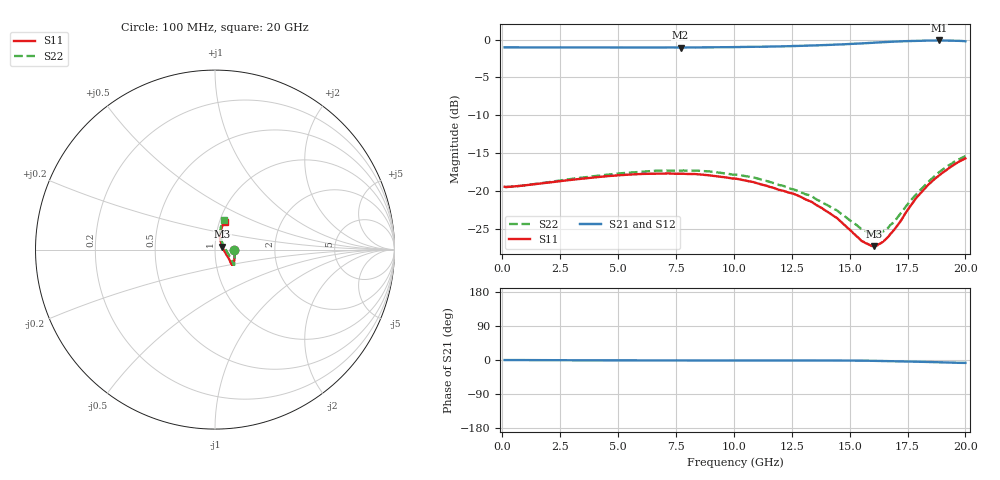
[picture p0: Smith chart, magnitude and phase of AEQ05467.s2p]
!Agilent Technologies,E8363B,MY43030965,A.07.50.67
!Agilent E8363B: A.07.50.67
!Date: Tuesday, August 27, 2013 09:58:20
!Correction: S11(Full 2 Port(1,2))
!S21(Full 2 Port(1,2))
!S12(Full 2 Port(1,2))
!S22(Full 2 Port(1,2))
!S2P File: Measurements: S11, S21, S12, S22:
# Hz S  dB  R 50
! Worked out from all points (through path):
!   3201 points, 100 MHz to 20 GHz, reference 50 ohm
!   highest |S21| = -0.11 dB at 18.86 GHz (marker M1); lowest = -1.0 dB at 7.699 GHz (marker M2)
!   lowest |S11| = -27.3 dB at 16.06 GHz (marker M3), VSWR 1.09, Z = 54.1 + j1.8 ohm
!   |S11| at or under -10 dB: start of sweep to end of sweep
!   |S22| runs from -25.7 to -15.4 dB; largest |S21 - S12| = 0.0079
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1e8  -19.44 -1.0  -1.02 -0.1  -1.02 -0.0  -19.48 -0.9
3.420812e9  -18.37 -26.0  -1.03 -0.7  -1.04 -0.8  -18.23 -26.0
5.162062e9  -17.89 -34.6  -1.04 -1.0  -1.04 -1.0  -17.64 -33.8
6.735406e9  -17.70 -39.2  -1.04 -1.2  -1.04 -1.3  -17.32 -37.7
7.699312e9  -17.71 -40.5  -1.05 -1.3  -1.06 -1.1  -17.30 -38.4
8.90575e9  -17.90 -41.5  -1.01 -1.3  -1.03 -1.2  -17.40 -38.7
1.005e10  -18.37 -40.7  -0.98 -1.3  -1.02 -1.0  -17.83 -37.5
1.098281e10  -18.95 -39.5  -0.94 -1.3  -0.95 -1.2  -18.31 -35.9
1.257481e10  -20.36 -33.9  -0.84 -1.2  -0.89 -0.8  -19.78 -29.7
1.337081e10  -21.46 -30.7  -0.78 -1.3  -0.78 -1.2  -20.69 -25.1
1.447775e10  -23.63 -20.8  -0.64 -1.3  -0.66 -1.2  -22.60 -14.9
1.555981e10  -26.67 3.2  -0.49 -1.8  -0.50 -1.6  -25.08 7.8
1.587075e10  -27.13 14.6  -0.44 -2.0  -0.45 -1.9  -25.60 17.6
1.605731e10  -27.28 22.6  -0.41 -2.2  -0.45 -2.0  -25.66 24.7
1.631228e10  -26.94 34.4  -0.36 -2.4  -0.37 -2.1  -25.53 34.7
1.668541e10  -25.98 48.7  -0.30 -2.7  -0.31 -2.4  -24.78 48.2
1.713316e10  -24.25 61.8  -0.24 -3.3  -0.25 -3.2  -23.21 61.0
1.79105e10  -20.80 71.7  -0.16 -4.5  -0.18 -4.4  -20.29 72.3
1.839556e10  -19.18 73.4  -0.12 -5.2  -0.15 -5.1  -18.79 75.1
1.886197e10  -17.94 73.2  -0.11 -6.1  -0.14 -6.0  -17.51 75.3
1.958334e10  -16.38 72.0  -0.14 -7.2  -0.19 -6.9  -16.01 74.7
2e10  -15.68 70.4  -0.22 -7.7  -0.22 -7.5  -15.40 73.7
